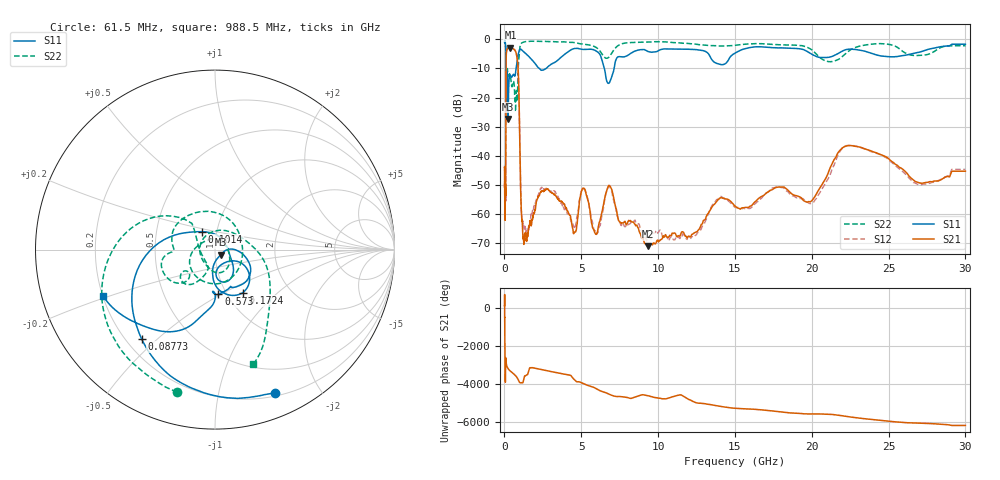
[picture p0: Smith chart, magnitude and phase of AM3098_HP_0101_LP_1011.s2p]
! Date/Time: Thu, Feb 28, 2019 8:36 AM
! Network Analyzer: Agilent Technologies E8364B Rev: A.07.50.67
! Sweep from 0.010 to 30.000 GHz, 1601 Points, Sweep Type: LOG
! Power Supply: 5.022 V, 0.002 A
# Hz S DB R 50
!freq MagS11 AngS11 MagS21 AngS21 MagS12 AngS12 MagS22 AngS22
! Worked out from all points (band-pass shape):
!   1601 points, 10 MHz to 30 GHz, reference 50 ohm
!   highest |S21| = -2.82 dB at 387.8 MHz (marker M1); lowest = -71.2 dB at 9.349 GHz (marker M2)
!   |S21| within 3 dB of the highest: 114.5 MHz to 807.3 MHz (692.8 MHz wide, 150 % of centre)
!   lowest |S11| = -27.4 dB at 236.3 MHz (marker M3), VSWR 1.09, Z = 53.2 - j3.1 ohm
!   |S11| at or under -10 dB: 97.45 MHz to 756.8 MHz (659.4 MHz wide, 154 % of centre); 2.273 GHz to 2.71 GHz (437.6 MHz wide, 17.6 % of centre); 6.503 GHz to 7.137 GHz (634.7 MHz wide, 9.31 % of centre)
!   |S22| runs from -24.9 to -0.6 dB; largest |S21 - S12| = 0.013
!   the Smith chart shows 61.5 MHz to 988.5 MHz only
!   S11 on the Smith chart (normalised r, x): 61.5 MHz: 0.23, -1.48; 87.73 MHz: 0.26, -0.45; 101.4 MHz: 0.85, +0.17; 172.4 MHz: 1.19, -0.62; 573 MHz: 0.91, -0.49; 988.5 MHz: 0.20, -0.19
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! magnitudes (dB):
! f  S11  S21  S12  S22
! 10 MHz  -0.4  -44.0  -43.4  -0.6
! 38.04 MHz  -0.5  -60.7  -58.6  -1.0
! 61.5 MHz  -1.3  -50.3  -51.1  -1.7
! 77.42 MHz  -2.1  -52.6  -54.9  -2.5
! 87.73 MHz  -3.8  -38.2  -38.3  -4.2
! 101.4 MHz  -18.2  -12.0  -12.0  -21.1
! 144.7 MHz  -17.5  -3.7  -3.7  -13.8
! 172.4 MHz  -10.9  -3.5  -3.4  -10.2
! 236.3 MHz  -27.4  -2.9  -2.9  -12.4
! 387.8 MHz  -12.4  -2.8  -2.8  -12.9
! 550.5 MHz  -12.2  -3.2  -3.2  -14.6
! 573 MHz  -12.0  -3.2  -3.2  -14.4
! 859.3 MHz  -6.3  -8.1  -8.1  -17.6
! 988.5 MHz  -3.4  -32.7  -32.7  -3.4
! 1.093 GHz  -3.5  -58.6  -58.2  -1.4
! 1.238 GHz  -4.2  -68.6  -64.0  -1.0
! 2.084 GHz  -8.9  -55.7  -55.0  -0.6
! 7.926 GHz  -5.8  -63.9  -63.6  -1.2
! 9.349 GHz  -4.2  -71.2  -68.3  -0.9
! 19.8 GHz  -4.5  -55.8  -56.4  -3.0
! 22.56 GHz  -3.4  -36.5  -36.5  -3.5
! 30 GHz  -1.7  -45.4  -44.8  -2.2
